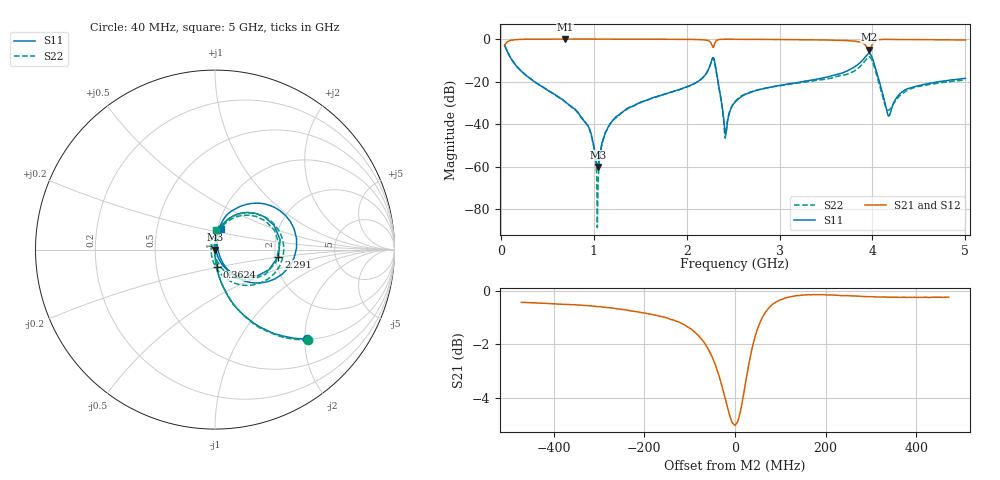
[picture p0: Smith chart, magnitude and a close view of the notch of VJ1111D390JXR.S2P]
! VJ1111D390JXR
! DATE 02/16/2022  11:06
! CAPACITORS MOUNTED IN SERIES ON 25 MIL THICK MICROSTRIP SUBSTRATE
# GHz  S  MA  R  50.00
!  FREQ  S11M  S11A  S21M  S21A  S12M  S12A  S22M  S22A
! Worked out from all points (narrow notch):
!   801 points, 40 MHz to 5 GHz, reference 50 ohm
!   highest |S21| = -0.01 dB at 691 MHz (marker M1); lowest = -5.0 dB at 3.965 GHz (marker M2)
!   notch at M2: 4.8 dB deep, 79.1 MHz wide at half that depth
!   lowest |S11| = -60.1 dB at 1.044 GHz (marker M3), VSWR 1.00, Z = 50.1 + j0.04 ohm
!   |S11| at or under -10 dB: 120.7 MHz to 2.269 GHz (2.149 GHz wide, 180 % of centre); 2.297 GHz to 3.892 GHz (1.595 GHz wide, 51.5 % of centre); 4.007 GHz to end of sweep
!   |S22| runs from -88.6 to -2.8 dB; largest |S21 - S12| = 0.039
!   S11 on the Smith chart (normalised r, x): 40 MHz: 1.00, -2.04; 362.4 MHz: 1.00, -0.20; 2.291 GHz: 2.08, -0.18; 5 GHz: 1.04, +0.24
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0.04  0.714 -44.4  0.6973 45.6  0.6984 45.7  0.7212 -44.3
0.133  0.2893 -73.4  0.9495 16.5  0.9659 18.0  0.293 -72.9
0.3624  0.09897 -84.7  0.9941 6.1  1.001 5.9  0.09973 -84.7
0.691  0.03397 -87.9  0.9985 2.8  1.004 2.6  0.03385 -89.5
0.8708  0.01409 -87.3  0.9979 1.9  1.002 1.9  0.01435 -90.6
0.97  0.006098 -88.0  0.9968 1.6  1.004 1.4  0.005898 -96.0
1.0444  0.0009899 23.8  0.9972 1.3  1.003 1.1  0.0002922 93.8
1.1002  0.00447 79.1  0.9965 1.2  1.003 0.9  0.004333 98.8
1.1932  0.01156 85.8  0.9957 0.9  1.003 0.7  0.01156 89.4
1.6954  0.0457 85.0  0.9907 -0.4  0.9974 -0.6  0.04545 86.3
2.1046  0.09594 80.2  0.9757 -2.7  0.9817 -2.9  0.09508 79.3
2.2472  0.2277 58.8  0.8807 -9.1  0.8864 -9.3  0.2236 55.7
2.2906  0.3553 -6.3  0.6532 9.2  0.6574 9.0  0.3474 -11.4
2.4146  0.005971 -12.4  0.9904 3.2  0.9958 3.0  0.004714 -174.3
2.52  0.03284 83.9  0.9879 1.3  0.9944 1.1  0.03437 97.8
3.3508  0.1094 79.8  0.962 -2.2  0.9677 -2.4  0.1036 83.0
3.8034  0.2197 68.8  0.895 -6.3  0.9008 -6.5  0.1771 67.8
3.9646  0.4585 7.8  0.561 5.3  0.564 5.2  0.3843 1.5
4.0142  0.2816 -41.2  0.8493 19.0  0.8549 18.8  0.2391 -54.8
4.1754  0.01553 13.0  0.9826 4.4  0.9897 4.2  0.02144 171.4
4.3614  0.06573 72.9  0.9729 1.6  0.9782 1.5  0.06015 111.3
5  0.1196 73.6  0.9506 -1.8  0.9569 -2.0  0.1097 88.1
